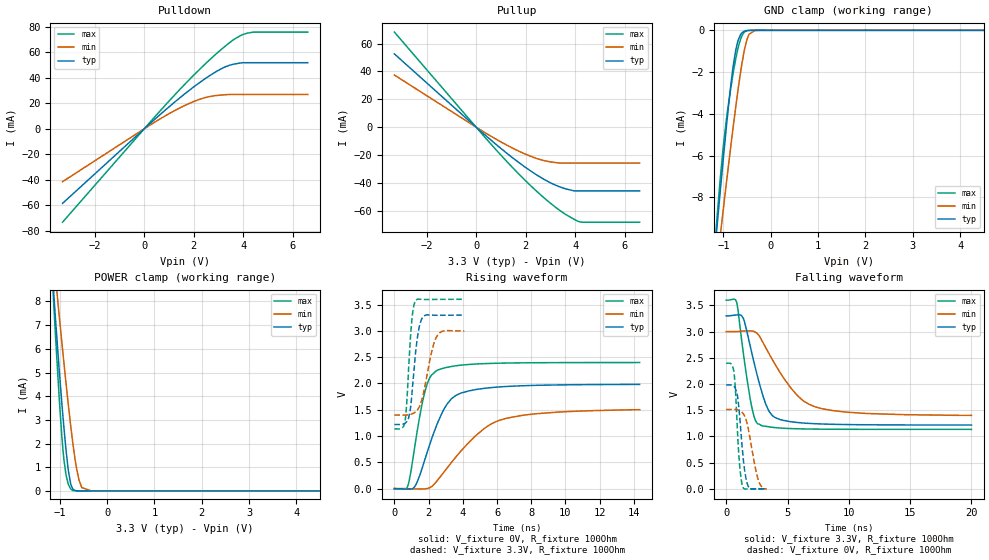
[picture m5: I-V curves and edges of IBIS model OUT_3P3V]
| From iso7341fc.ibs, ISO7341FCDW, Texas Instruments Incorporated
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|   OUT_3P3V Model
[Model]   OUT_3P3V
Model_type   3-state
Polarity   Non-Inverting
Vmeas = 1.65
Vref = 0
Cref = 15pF
Rref = 150
|   typ   min   max
|   (nom PVT)   (fast PVT)   (slow PVT)
C_comp   4.694e-13   2.619e-13   5.189e-13
| Where   Nom PVT is Nominal Process, 3.3V, 27C
|   Fast PVT is Strong Process, 3.6V, -40C
|   Slow PVT is Weak Process, 3.0V, 150C
[Voltage Range]   3.3   3   3.6
[Temperature Range]   27   150   -40
[Pullup Reference]   3.3   3   3.6
[Pulldown Reference]   0   0   0
[Power Clamp Reference]   3.3   3   3.6
[GND Clamp Reference]   0   0   0
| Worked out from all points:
|   slope of the pulldown table from 0 to 0.495 V, typ, clamps not added: 57 ohm
|   slope of the pullup table from 0 to 0.495 V, typ, clamps not added: 64.2 ohm
|   GND clamp passes 1 mA (typ) near -0.74 V on its own axis
|   POWER clamp passes 1 mA (typ) near -0.83 V on its own axis
|   falling waveform, V_fixture 3.3V, R_fixture 100Ohm: 20-80 % time 1.39ns typ, 2.82ns min, 910ps max; typ from 3.3 V to 1.22 V
|   rising waveform, V_fixture 0V, R_fixture 100Ohm: 20-80 % time 1.41ns typ, 2.65ns min, 809ps max; typ from 0 V to 1.98 V
|   rising waveform, V_fixture 3.3V, R_fixture 100Ohm: 20-80 % time 374ps typ, 613ps min, 273ps max; typ from 1.22 V to 3.3 V
|   falling waveform, V_fixture 0V, R_fixture 100Ohm: 20-80 % time 461ps typ, 732ps min, 338ps max; typ from 1.98 V to 0 V
[Pulldown]
|   Voltage   I(typ)   I(min)   I(max)
-3.3V     -58.55mA   -41.56mA   -73.33mA
63mV      1.121mA    792.5uA    1.405mA
1.251V    21.35mA    14.53mA    27.05mA
1.945V    32.11mA    20.99mA    41.09mA
2.424V    38.88mA    24.29mA    50.23mA
3.049V    46.5mA     26.38mA    61.3mA
3.422V    49.72mA    26.9mA     67.27mA
3.914V    51.72mA    26.92mA    73.45mA
4.396V    51.85mA    26.92mA    75.88mA
6.6V      51.85mA    26.92mA    75.88mA
[GND Clamp]
|   Voltage   I(typ)   I(min)   I(max)
-3.3V     -66.33mA   -55.51mA   -79.32mA
-1.154V   -9.888mA   -11.57mA   -9.535mA
-1.132V   -9.323mA   -11.12mA   -8.884mA
-1.075V   -7.914mA   -9.997mA   -7.314mA
-1.003V   -6.166mA   -8.588mA   -5.556mA
-916.8mV  -4.163mA   -6.923mA   -3.914mA
-790.8mV  -1.668mA   -4.577mA   -2.014mA
-686.4mV  -466.9uA   -2.773mA   -810uA
-552mV    -35.48uA   -889.3uA   -75.75uA
-459mV    -3.256uA   -186.3uA   -4.948uA
-312mV    -39.18nA   -4.457uA   -22.52nA
6.6V      0A         0A         0A
[Pullup]
|   Voltage   I(typ)   I(min)   I(max)
-3.3V     52.57mA    37.4mA     68.21mA
63mV      -997.5uA   -703.4uA   -1.301mA
1.045V    -15.93mA   -11.03mA   -20.93mA
1.647V    -24.35mA   -16.58mA   -32.23mA
2.391V    -33.65mA   -22.14mA   -45.15mA
2.826V    -38.29mA   -24.32mA   -52.02mA
3.231V    -41.81mA   -25.45mA   -57.81mA
3.634V    -44.37mA   -25.78mA   -62.81mA
3.963V    -45.73mA   -25.78mA   -66.21mA
4.161V    -45.73mA   -25.78mA   -67.86mA
6.6V      -45.73mA   -25.78mA   -68.17mA
[POWER Clamp]
|   Voltage   I(typ)   I(min)   I(max)
-3.3V     77.67mA    63.46mA    93.35mA
-1.191V   10.23mA    11.25mA    10.25mA
-1.101V   7.578mA    9.276mA    6.957mA
-1.01V    5.085mA    7.382mA    3.893mA
-956.4mV  3.722mA    6.289mA    2.325mA
-912mV    2.681mA    5.41mA     1.329mA
-815.1mV  818.2uA    3.574mA    265.2uA
-732mV    107.8uA    2.152mA    26.5uA
-594mV    1.601uA    459.7uA    296.2nA
-534mV    273.1nA    139.4uA    34.96nA
-330mV    0A         698.2nA    0A
6.6V      0A         0A         0A
[Ramp]
R_load = 100
|   typ   min   max
dV/dt_r   1.18945/1.40757e-09   0.907414/2.69185e-09   1.43821/8.05471e-10
dV/dt_f   1.24916/1.39303e-09   0.958553/2.81399e-09   1.47894/9.09238e-10
[Falling Waveform]
V_fixture = 3.3V
V_fixture_min = 3V
V_fixture_max = 3.6V
R_fixture = 100Ohm
|   Time   V(typ)   V(min)   V(max)
0s        3.3V       3V         3.6V
850ps     3.318V     3.001V     3.562V
1.4ns     3.251V     3.01V      2.583V
1.956ns   2.727V     3.014V     1.717V
2.588ns   2.113V     2.95V      1.24V
3.234ns   1.609V     2.689V     1.193V
3.752ns   1.401V     2.471V     1.175V
5.734ns   1.268V     1.798V     1.147V
7.192ns   1.244V     1.57V      1.141V
20ns      1.218V     1.402V     1.135V
[Rising Waveform]
V_fixture = 0V
V_fixture_min = 0V
V_fixture_max = 0V
R_fixture = 100Ohm
|   Time   V(typ)   V(min)   V(max)
0s        509.2pV    2.809nV    468.6pV
776ps     -9.281mV   -1.12mV    42.84mV
1.198ns   41.41mV    -5.062mV   810.9mV
1.784ns   554mV      -4.479mV   1.844V
2.106ns   876.9mV    23.62mV    2.127V
2.542ns   1.261V     167mV      2.256V
3.554ns   1.763V     585.6mV    2.333V
4.828ns   1.887V     1.028V     2.37V
6.152ns   1.933V     1.299V     2.385V
14.34ns   1.981V     1.5V       2.397V
[Rising Waveform]
V_fixture = 3.3V
V_fixture_min = 3V
V_fixture_max = 3.6V
R_fixture = 100Ohm
|   Time   V(typ)   V(min)   V(max)
0s        1.218V     1.398V     1.136V
616ps     1.241V     1.398V     1.253V
712ps     1.268V     1.399V     1.582V
836ps     1.349V     1.404V     2.31V
996ps     1.692V     1.416V     3.111V
1.232ns   2.567V     1.459V     3.574V
1.616ns   3.237V     1.701V     3.596V
2.192ns   3.298V     2.615V     3.596V
2.512ns   3.295V     2.91V      3.597V
4.082ns   3.298V     2.996V     3.599V
[Falling Waveform]
V_fixture = 0V
V_fixture_min = 0V
V_fixture_max = 0V
R_fixture = 100Ohm
|   Time   V(typ)   V(min)   V(max)
0s        1.982V     1.515V     2.397V
626ps     1.959V     1.516V     2.238V
752ps     1.911V     1.515V     1.895V
916ps     1.776V     1.511V     1.116V
1.062ns   1.471V     1.501V     541.3mV
1.342ns   695.1mV    1.449V     43.22mV
1.6ns     214.3mV    1.335V     -2.44mV
1.828ns   34.49mV    1.111V     1.029mV
2.578ns   1.175mV    200.8mV    1.342mV
3.3ns     2.859uV    18.32uV    446.2nV
